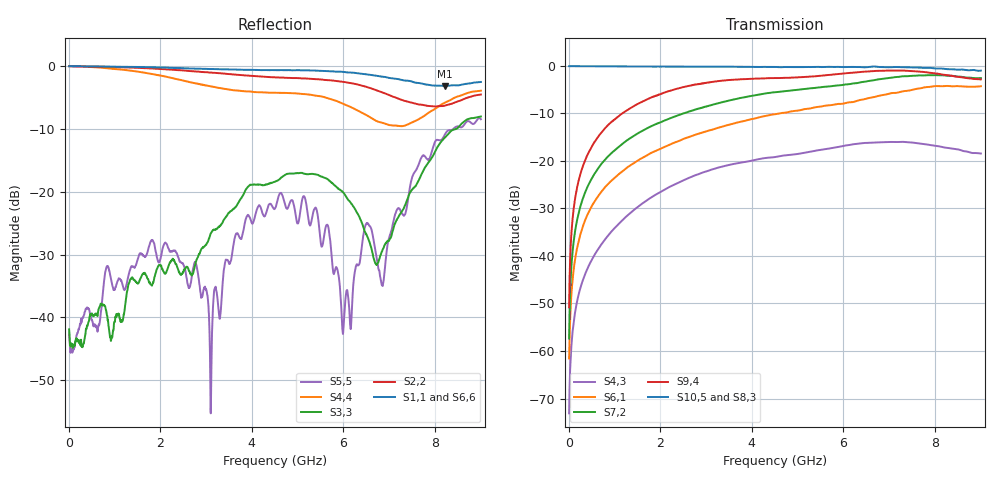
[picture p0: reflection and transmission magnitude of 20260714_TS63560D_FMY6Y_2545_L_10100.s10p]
# GHz S DB R 50
! CMT, SN0916, 25263762, 26.7.0
! Date: 15.07.2026 13:44:18
! Data: Format
! Freq S1.1:dB/Ang S1.2:dB/Ang S1.3:dB/Ang S1.4:dB/Ang S1.5:dB/Ang S1.6:dB/Ang S1.7:dB/Ang S1.8:dB/Ang S1.9:dB/Ang S1.10:dB/Ang
!  S2.1:dB/Ang S2.2:dB/Ang S2.3:dB/Ang S2.4:dB/Ang S2.5:dB/Ang S2.6:dB/Ang S2.7:dB/Ang S2.8:dB/Ang S2.9:dB/Ang S2.10:dB/Ang
!  S3.1:dB/Ang S3.2:dB/Ang S3.3:dB/Ang S3.4:dB/Ang S3.5:dB/Ang S3.6:dB/Ang S3.7:dB/Ang S3.8:dB/Ang S3.9:dB/Ang S3.10:dB/Ang
!  S4.1:dB/Ang S4.2:dB/Ang S4.3:dB/Ang S4.4:dB/Ang S4.5:dB/Ang S4.6:dB/Ang S4.7:dB/Ang S4.8:dB/Ang S4.9:dB/Ang S4.10:dB/Ang
!  S5.1:dB/Ang S5.2:dB/Ang S5.3:dB/Ang S5.4:dB/Ang S5.5:dB/Ang S5.6:dB/Ang S5.7:dB/Ang S5.8:dB/Ang S5.9:dB/Ang S5.10:dB/Ang
!  S6.1:dB/Ang S6.2:dB/Ang S6.3:dB/Ang S6.4:dB/Ang S6.5:dB/Ang S6.6:dB/Ang S6.7:dB/Ang S6.8:dB/Ang S6.9:dB/Ang S6.10:dB/Ang
!  S7.1:dB/Ang S7.2:dB/Ang S7.3:dB/Ang S7.4:dB/Ang S7.5:dB/Ang S7.6:dB/Ang S7.7:dB/Ang S7.8:dB/Ang S7.9:dB/Ang S7.10:dB/Ang
!  S8.1:dB/Ang S8.2:dB/Ang S8.3:dB/Ang S8.4:dB/Ang S8.5:dB/Ang S8.6:dB/Ang S8.7:dB/Ang S8.8:dB/Ang S8.9:dB/Ang S8.10:dB/Ang
!  S9.1:dB/Ang S9.2:dB/Ang S9.3:dB/Ang S9.4:dB/Ang S9.5:dB/Ang S9.6:dB/Ang S9.7:dB/Ang S9.8:dB/Ang S9.9:dB/Ang S9.10:dB/Ang
!  S10.1:dB/Ang S10.2:dB/Ang S10.3:dB/Ang S10.4:dB/Ang S10.5:dB/Ang S10.6:dB/Ang S10.7:dB/Ang S10.8:dB/Ang S10.9:dB/Ang S10.10:dB/Ang
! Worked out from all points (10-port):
!   2001 points, 10 MHz to 9 GHz, reference 50 ohm
!   strongest paths, dB at 10 MHz, 2.257 GHz, 4.505 GHz, 6.753 GHz, 9 GHz:
!     S10,5: -0.1, -0.2, -0.2, -0.2, -1.0
!     S8,3: -0.1, -0.2, -0.4, -0.4, -1.3
!     S9,4: -50.8, -5.1, -2.6, -1.1, -2.8
!     S7,2: -57.4, -10.9, -5.5, -2.9, -2.6
!     S6,1: -61.6, -16.4, -10.2, -6.3, -4.3
!     S4,3: -73.1, -25.2, -19.2, -16.1, -18.4
!   lowest |S11| = -3.2 dB at 8.209 GHz (marker M1), VSWR 5.56, Z = 11.1 - j23.6 ohm
!   |S11| at or under -10 dB: nowhere
